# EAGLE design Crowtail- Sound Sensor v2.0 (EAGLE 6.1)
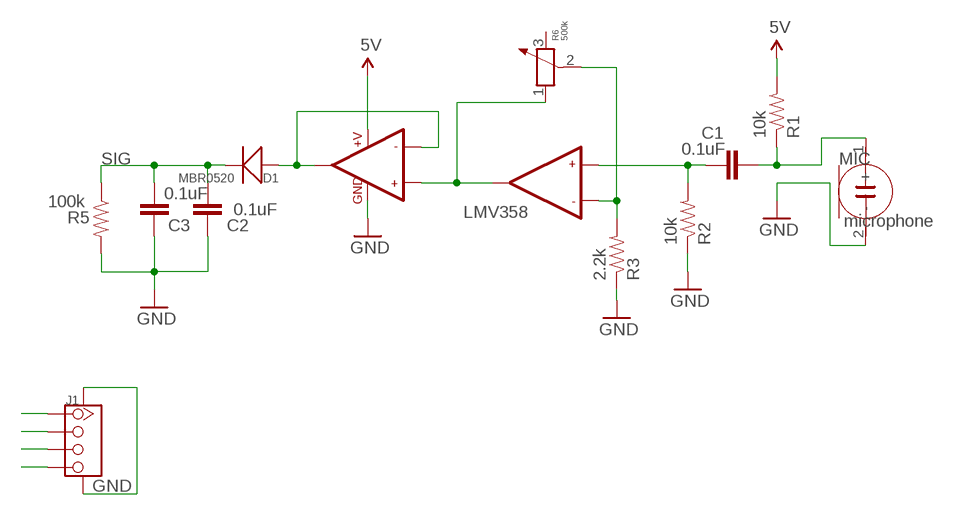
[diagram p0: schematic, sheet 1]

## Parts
C1  0.1uF  CAP0603-CAP  [0603-CAP]
C2  0.1uF  CAP0603-CAP  [0603-CAP]
C3  0.1uF  CAP0603-CAP  [0603-CAP]
D1  MBR0520  D'MBR0520LT1'  [SOD123-2.7X1.6]
J1  TWIG-4P-2.0-SMD-FEMALE-REINFORCE'90D'  [4P-SMD-2.0-90D]
MIC  microphone  MICROPHONE  [2P-D8.9MM]
R1  10k  RESISTOR0603-RES  [0603-RES]
R2  10k  RESISTOR0603-RES  [0603-RES]
R3  2.2k  RESISTOR0603-RES  [0603-RES]
R5  100k  RESISTOR0603-RES  [0603-RES]
R6  500k  R-POTENTIOMETER-SMD  [3P-SMD-SQUA-3.6X3.3]
U1  LMV358  [SO08]

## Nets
5V: J1.3 R1.2 U1.8(+V)
GND: C2.1 C3.1 J1.4 J1.SS1 J1.SS2 MIC.2(-) R2.1 R3.1 R5.2 U1.4(GND)
N$6: C1.1 MIC.1(+) R1.1
N$8: R3.2 R6.2 U1.6(-IN2)
N$11: C1.2 R2.2 U1.5(+IN2)
N$13: D1.2(+) U1.1(OUT1) U1.2(-IN1)
N$16: R6.1 U1.3(+IN1) U1.7(OUT2)
NC: J1.2
SIG: C2.2 C3.2 D1.1(-) J1.1 R5.1
Unconnected: R6.3

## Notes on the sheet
- LMV358

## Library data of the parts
C1-C3 = SparkFun:CAP: Capacitor
D1 = Discrete:D*
J1 = Connector:TWIG-4P-2.0-SMD-FEMALE-REINFORCE
MIC = template:MICROPHONE
R1-R3 R5 = SparkFun:RESISTOR: Resistor
R6 = Discrete:R-POTENTIOMETER*: Potentiometer
U1 = SparkFun:LMV358

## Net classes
0 default: width 0.203 mm, drill 0.305 mm, clearance 0.203 mm
1 power: width 0.254 mm

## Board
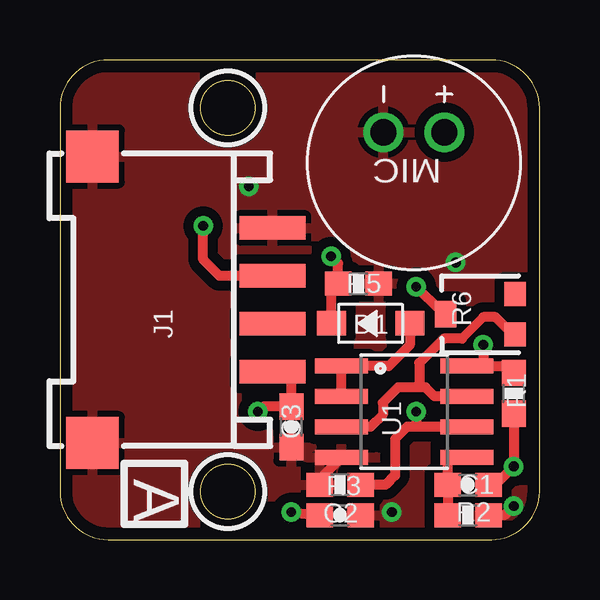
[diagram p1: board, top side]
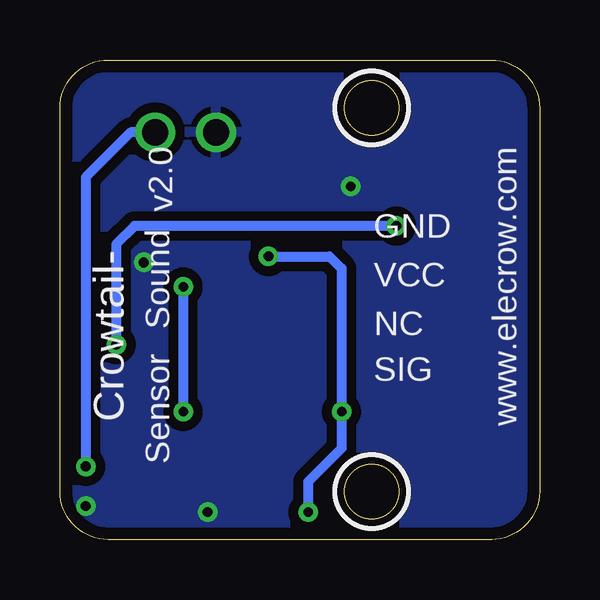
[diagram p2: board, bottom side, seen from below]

Size 20 x 20 mm. Coordinates in mm from the lower left corner, seen from the top.
Outline: 20,2 20,18 arc90 18,20 2,20 arc90 0,18 0,2 arc90 2,0 18,0 arc90 20,2
Outline: circle at 7,18 radius 1.14
Outline: circle at 7,2 radius 1.14
Copper layers (1*16): Top 0.035mm / dielectric 1.5mm / Bottom 0.035mm
Design rules "default *": minimum track width 10mil, minimum drill 10mil, track to track 8mil, track to pad 8mil, pad to pad 8mil, via to via 8mil, smd to smd 0mil, copper to edge 20mil, drill to drill 8mil, minimum pad ring 10mil, minimum via ring 8mil, stop-mask expansion 2mil, vias tented up to drill 100mil, thermal gap 10mil
tRestrict: area -4.6,15.6 to -1.6,18.6; area -5.7,8.2 to -2.7,11.3
bRestrict: area -4.6,15.6 to -1.6,18.6; area -5.7,8.2 to -2.7,11.3

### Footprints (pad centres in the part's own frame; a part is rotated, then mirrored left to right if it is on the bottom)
0603-CAP = smd 1.1 x 1: 1 -0.85,0; 2 0.85,0
SOD123-2.7X1.6 = smd 1.2 x 1.02: 1 1.635,0; 2 -1.635,0
4P-SMD-2.0-90D = smd 0.965 x 2.74: 1 -3,-0.1; 2 -1,-0.1; 3 1,-0.1; 4 3,-0.1 | smd 2.159 x 2.184: SS1 -5.974,7.4; SS2 5.974,7.4
2P-D8.9MM = drill 1.1: 1 -1.27,1.27; 2 -1.27,-1.27
0603-RES = smd 1.1 x 1: 1 -0.85,0; 2 0.85,0
3P-SMD-SQUA-3.6X3.3 = smd 1 x 0.9: 1 -0.85,-1.45; 3 0.85,-1.45 | smd 1.1 x 0.9: 2 0,1.45
SO08 = smd 0.61 x 2.21: 1 -1.905,-2.616; 2 -0.635,-2.616; 3 0.635,-2.616; 4 1.905,-2.616; 5 1.905,2.616; 6 0.635,2.616; 7 -0.635,2.616; 8 -1.905,2.616

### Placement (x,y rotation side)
C1  17.02,2.29 180 top
C2  11.68,1.02 180 top
C3  9.65,4.7 90 top
D1  12.95,9.02 180 top
J1  8.76,10 90 top
MIC  14.76,15.71 270 top
R1  18.92,6.1 90 top
R2  17.02,1.02 180 top
R3  11.68,2.29 0 top
R5  12.45,10.67 0 top
R6  17.53,9.4 90 top
U1  14.35,5.33 270 top

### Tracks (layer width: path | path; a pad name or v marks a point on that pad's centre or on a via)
5V  (via drill 0.41)
  Top 0.406: U1.8 17.65,7.24 | 17.65,7.24 18.63,7.24 R1.2 | J1.3 6.65,11 5.97,11.68 v5.97,13.08 | v17.65,8.13 17.65,7.24
  Bottom 0.406: v5.97,13.08 16.89,13.08 17.65,12.32 v17.65,8.13
GND  (via drill 0.41)
  Top 0.406: R3.1 10.83,2.53 U1.4 | v18.92,1.4 18.54,1.02 17.91,1.02
  other vias: 7.87,14.73 13.84,1.14 16.51,11.56
  pour Top (isolate 0.406): -1.27,20.32 20.32,20.32 20.32,0 -1.27,0
  pour Bottom (isolate 0.406): -1.27,20.32 20.32,20.32 20.32,0 -1.27,0
N$6  (via drill 0.41)
  Top 0.406: C1.1 18.16,2.29 v18.92,3.05 R1.1
  Bottom 0.406: MIC.1 17.05,16.98 18.92,15.11 v18.92,3.05
N$8  (via drill 0.4, 0.41)
  Top 0.406: U1.6 14.86,4.7 | 14.86,4.7 14.48,4.7 13.97,4.19 13.97,2.67 13.59,2.29 R3.2 | R6.2 15.88,9.53 v14.86,10.54 | v14.86,5.33 14.86,4.7
  Bottom 0.406: v14.86,10.54 v14.86,5.33
N$11
  Top 0.406: R2.2 C1.2 16.17,3.39 16.13,3.43 U1.5
N$13
  Top 0.406: U1.2 U1.1 13.72,7.24 14.59,8.11 D1.2
N$16
  Top 0.356: 17.65,9.27 16.76,8.38
  Top 0.406: U1.7 15.62,5.97 15.24,6.35 14.99,6.35 | 14.99,6.35 14.1,6.35 13.46,5.71 13.46,5.21 12.95,4.7 U1.3 | 14.99,6.35 14.99,7.37 16,8.38 16.76,8.38 | R6.1 19.14,8.68 18.76,8.68 18.16,9.27 17.65,9.27
SIG  (via drill 0.4, 0.41)
  Top 0.406: J1.1 8.97,7.11 9.53,7.11 9.65,6.99 C3.2 8.47,5.55 v8.26,5.33 | v9.65,1.14 C2.2 | D1.1 11.32,10.39 R5.1 11.6,11.52 v11.3,11.81
  Bottom 0.406: v9.65,1.14 9.65,2.41 8.26,3.81 v8.26,5.33 8.26,11.3 8.76,11.81 v11.3,11.81

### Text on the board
tPlace: A
bPlace: www.elecrow.com | v2.0 | GND | Sound | Crowtail- | VCC | NC | Sensor | SIG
